(* Logix 5000 AddOnInstructionDefinition export YAI_Assy_72_73_20_21_EIP_Hz; software revision 17.00 *)

ADD_ON_INSTRUCTION YAI_Assy_72_73_20_21_EIP_Hz   (* revision 1.0, vendor Yaskawa America, Inc. *)
// YAI Assembly 72/73 and 20/21
// Speed is given in Hz
// Torque is given in % rated torque
// Help:
// This add-on instruction is for use with input assemblie 72 or 73 and output assemblies 22 or 23.
// Node_Input_Assy is defined as the node's input assembly integer array.
// Node_Output_Assy is defined as the node's output assembly integer array.
// Torque limit/reference and torque output variables are only available with A1000.
VAR_IN_OUT
   Node_Input_Assy : AB:ETHERNET_MODULE_INT_6Bytes:I:0; {required}   // Input assembly words
   Node_Output_Assy : AB:ETHERNET_MODULE_INT_4Bytes:O:0; {required}   // Output assembly words
END_VAR
VAR_INPUT
   RunFwd : BOOL; {visible}   // Forward run command
   RunRev : BOOL; {visible}   // Reverse run command
   FaultReset : BOOL; {visible}   // Fault reset command
   Net_Control : BOOL;   // Network control bit to switch between b1-02 setting and network.
   Net_Ref : BOOL;   // Network reference bit to switch between b1-01 setting and network.
   Freq_Ref : REAL; {visible}   // Frequency reference command in Hz (xx.xx resolution)
END_VAR
VAR_OUTPUT
   Faulted : BOOL; {visible}   // Drive faulted status bit
   Warning : BOOL; {visible}   // Drive warning (alarm) status bit
   RunningFwd : BOOL; {visible}   // Drive running forward status bit
   RunningRev : BOOL; {visible}   // Drive running reverse status bit
   Ready : BOOL; {visible}   // Drive ready status bit
   NetRefStatus : BOOL; {visible}   // Drive network reference status bit (1 = reference coming from network)
   NetCtrlStatus : BOOL; {visible}   // Drive network run source status bit (1 = source coming from network)
   Drive_State : INT;   // Drive Status - Refer to class 0x29, Instance 0x1, Attribute 0x6 for details
   At_Speed : BOOL; {visible}   // Drive at commanded speed status bit
   Output_Freq : REAL; {visible}   // Drive output frequency in Hz (xx.xx resolution)
   Torque_Actual : REAL; {visible}   // Drive torque output in engineering units.
END_VAR
VAR_INPUT
   Motor_Rated_Torq : REAL;
END_VAR
VAR
   FRef_Convert : DINT;
   FOut_Convert : REAL;
   FOut_Temp : REAL;
   DriveStatusTempBits : INT;
   TOut_Convert : REAL;
   TOut_Temp : REAL;
   Tout_Convert_Temp : REAL;
END_VAR

ROUTINE Logic   (* ladder *)
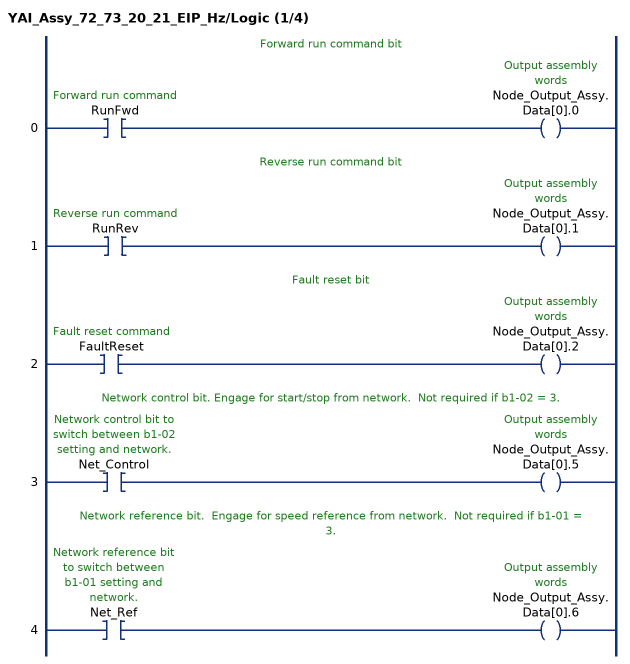
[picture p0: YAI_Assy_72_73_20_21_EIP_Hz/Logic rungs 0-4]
   // Forward run command bit
   0: XIC(RunFwd)OTE(Node_Output_Assy.Data[0].0);
   // Reverse run command bit
   1: XIC(RunRev)OTE(Node_Output_Assy.Data[0].1);
   // Fault reset bit
   2: XIC(FaultReset)OTE(Node_Output_Assy.Data[0].2);
   // Network control bit. Engage for start/stop from network.  Not required if b1-02 = 3.
   3: XIC(Net_Control)OTE(Node_Output_Assy.Data[0].5);
   // Network reference bit.  Engage for speed reference from network.  Not required if b1-01 = 3.
   4: XIC(Net_Ref)OTE(Node_Output_Assy.Data[0].6);
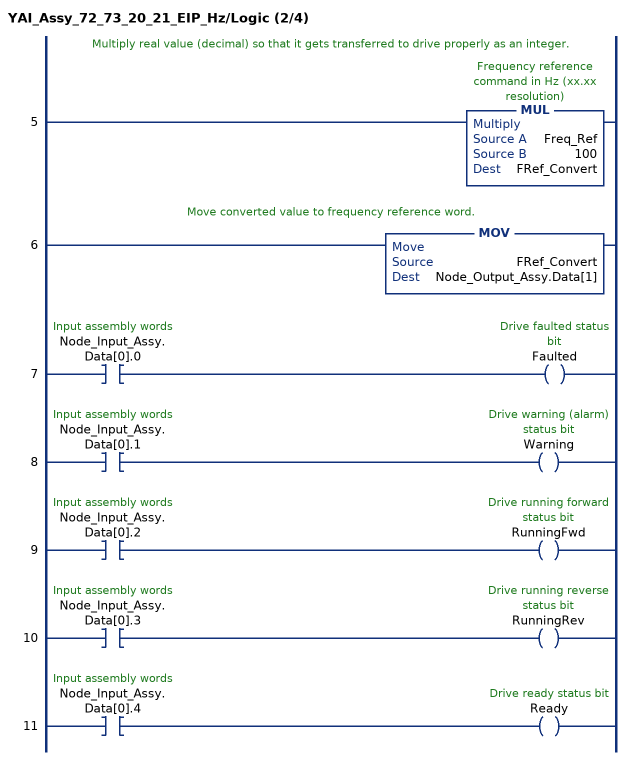
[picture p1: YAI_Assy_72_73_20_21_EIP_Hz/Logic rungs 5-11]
   // Multiply real value (decimal) so that it gets transferred to drive properly as an integer.
   5: MUL(Freq_Ref,100,FRef_Convert);
   // Move converted value to frequency reference word.
   6: MOV(FRef_Convert,Node_Output_Assy.Data[1]);
   7: XIC(Node_Input_Assy.Data[0].0)OTE(Faulted);
   8: XIC(Node_Input_Assy.Data[0].1)OTE(Warning);
   9: XIC(Node_Input_Assy.Data[0].2)OTE(RunningFwd);
   10: XIC(Node_Input_Assy.Data[0].3)OTE(RunningRev);
   11: XIC(Node_Input_Assy.Data[0].4)OTE(Ready);
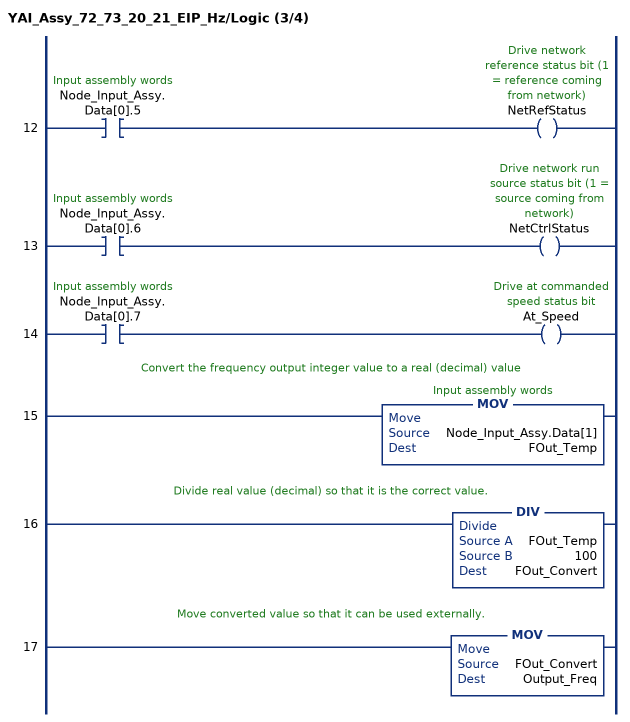
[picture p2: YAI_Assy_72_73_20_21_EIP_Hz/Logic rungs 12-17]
   12: XIC(Node_Input_Assy.Data[0].5)OTE(NetRefStatus);
   13: XIC(Node_Input_Assy.Data[0].6)OTE(NetCtrlStatus);
   14: XIC(Node_Input_Assy.Data[0].7)OTE(At_Speed);
   // Convert the frequency output integer value to a real (decimal) value
   15: MOV(Node_Input_Assy.Data[1],FOut_Temp);
   // Divide real value (decimal) so that it is the correct value.
   16: DIV(FOut_Temp,100,FOut_Convert);
   // Move converted value so that it can be used externally.
   17: MOV(FOut_Convert,Output_Freq);
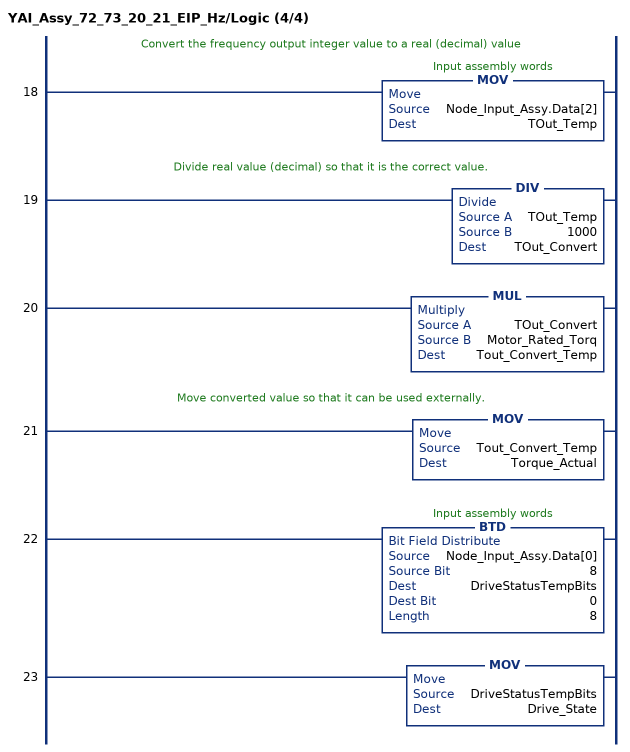
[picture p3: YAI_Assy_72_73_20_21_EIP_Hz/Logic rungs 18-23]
   // Convert the frequency output integer value to a real (decimal) value
   18: MOV(Node_Input_Assy.Data[2],TOut_Temp);
   // Divide real value (decimal) so that it is the correct value.
   19: DIV(TOut_Temp,1000,TOut_Convert);
   20: MUL(TOut_Convert,Motor_Rated_Torq,Tout_Convert_Temp);
   // Move converted value so that it can be used externally.
   21: MOV(Tout_Convert_Temp,Torque_Actual);
   22: BTD(Node_Input_Assy.Data[0],8,DriveStatusTempBits,0,8);
   23: MOV(DriveStatusTempBits,Drive_State);
END_ROUTINE
END_ADD_ON_INSTRUCTION
